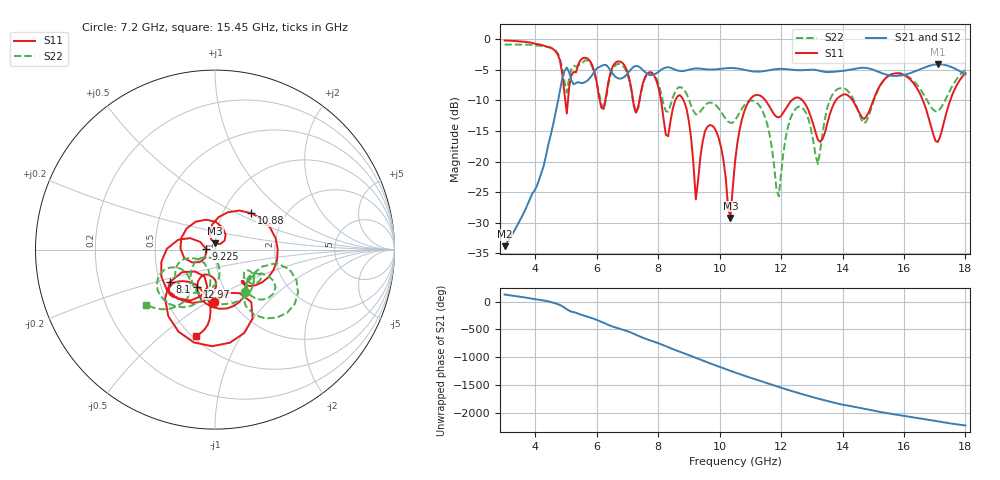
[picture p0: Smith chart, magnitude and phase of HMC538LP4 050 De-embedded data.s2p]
! Chelmsford, MA 01824
! http://www.hittite.com
! Tel: 978-250-3343
! Fax: 978-250-3373
! Device  :  HMC538LP4
! Description:  600 Analog Phase Shifter
! Frequency  :  6.0 GHz - 15.0 GHz
! Package  :  LP4  - 4x4 mm Quad Flatpack No-Lead (QFN) Plastic Package: 24 pin
! Ports  :  2 RF, 1 DC
!  Pin  3  = Rfin  = Port 1
!  Pin  16  = Rfout = Port 2
!  pin  21  = vCTL
! Voltages:  VCTL  = 0 to 5.0 Volts
! Currents :  Vb(V)  Vd(V)  Ib(mA)  Id(mA)
!  0.00  5.00  0.000000	0.476943
! Data:  The device was measured on evaluation board 111296-1.
!  Data was collected using a calibrated network analyzer.
!  The evaluation circuit board was modeled and simulated.This was use
!  to removed the evaluation board circuit from the measured data.
!  The reference plane is the center of the package pin.
! Misc:  Lot #
!Date Measured:  03 - 11 -2009
! Date:  03 - 17 -2009
! Note:
!  Hittite Microwave supplies this data as a sample of measured data at the
!  package pin for this package product.  Your particular data for this product
!  may vary.
!  Data was taken at 25 degrees C.
!  Hittite Microwave reserves the right to change this data at anytime.
# MHz S MA R 50
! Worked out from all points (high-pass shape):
!   201 points, 3 GHz to 18 GHz, reference 50 ohm
!   highest |S21| = -4.09 dB at 17.1 GHz (marker M1); lowest = -33.8 dB at 3 GHz (marker M2)
!   |S21| within 3 dB of the highest: 4.851 GHz to 5.218 GHz (367.1 MHz wide, 7.29 % of centre); 5.576 GHz to end of sweep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
!   lowest |S11| = -29.2 dB at 10.35 GHz (marker M3), VSWR 1.07, Z = 50 + j3.46 ohm
!   |S11| at or under -10 dB: 8.824 GHz to 10.97 GHz (2.146 GHz wide, 21.7 % of centre); 12.7 GHz to 13.78 GHz (1.085 GHz wide, 8.2 % of centre); 16.62 GHz to 17.51 GHz (891.7 MHz wide, 5.23 % of centre)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
!   |S22| runs from -25.7 to -0.9 dB; largest |S21 - S12| = 0.0025
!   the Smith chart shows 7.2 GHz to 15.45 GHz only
!   S11 on the Smith chart (normalised r, x): 7.2 GHz: 0.83, -0.54; 8.1 GHz: 0.57, -0.23; 9.225 GHz: 0.91, +0.01; 10.88 GHz: 1.35, +0.60; 12.97 GHz: 0.76, -0.33; 15.45 GHz: 0.52, -0.66
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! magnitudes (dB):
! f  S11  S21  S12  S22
! 3 GHz  -0.2  -33.8  -33.9  -0.9
! 4.65 GHz  -1.9  -12.3  -12.3  -1.8
! 5.025 GHz  -12.1  -4.6  -4.6  -8.7
! 5.55 GHz  -3.1  -7.1  -7.2  -3.8
! 7.2 GHz  -10.6  -4.5  -4.5  -10.8
! 8.025 GHz  -8.2  -5.3  -5.3  -7.5
! 8.1 GHz  -10.2  -5.0  -5.0  -8.9
! 8.85 GHz  -10.3  -5.2  -5.2  -8.3
! 9.225 GHz  -26.2  -4.8  -4.8  -12.3
! 9.75 GHz  -14.1  -4.9  -5.0  -10.4
! 10.35 GHz  -29.2  -4.7  -4.7  -13.7
! 10.5 GHz  -20.1  -4.7  -4.7  -13.2
! 10.88 GHz  -10.9  -5.1  -5.1  -10.4
! 11.47 GHz  -9.9  -5.2  -5.2  -12.7
! 11.93 GHz  -12.8  -4.8  -4.8  -25.7
! 12.38 GHz  -9.9  -5.0  -5.0  -12.1
! 12.97 GHz  -12.8  -5.0  -5.0  -14.7
! 13.05 GHz  -14.0  -5.0  -5.0  -16.7
! 15.45 GHz  -6.2  -5.8  -5.8  -6.2
! 15.53 GHz  -5.9  -5.9  -5.9  -5.9
! 17.1 GHz  -16.8  -4.1  -4.1  -11.8
! 18 GHz  -5.5  -5.7  -5.7  -5.0
